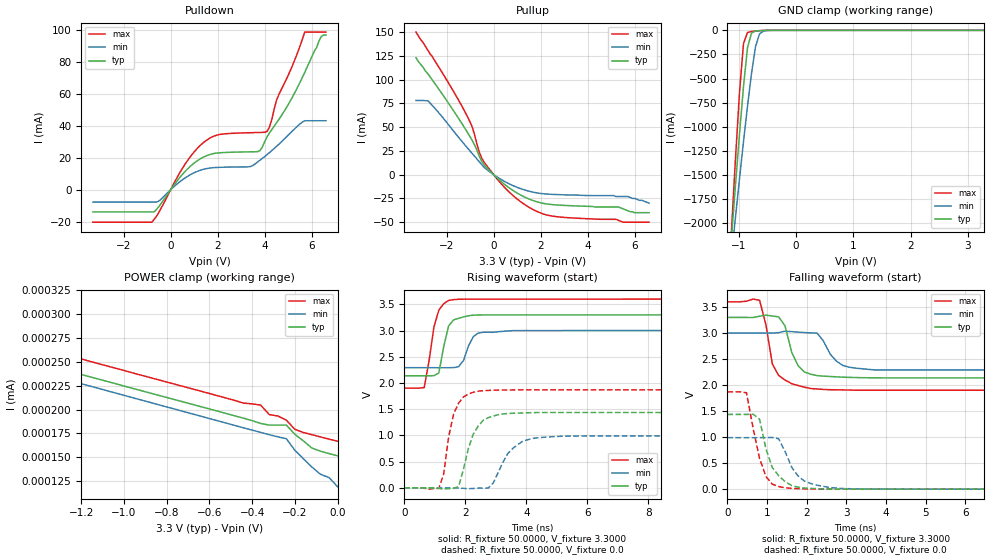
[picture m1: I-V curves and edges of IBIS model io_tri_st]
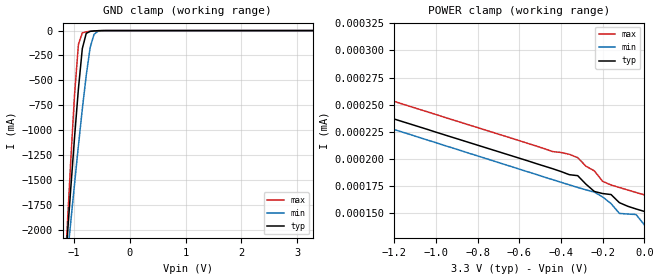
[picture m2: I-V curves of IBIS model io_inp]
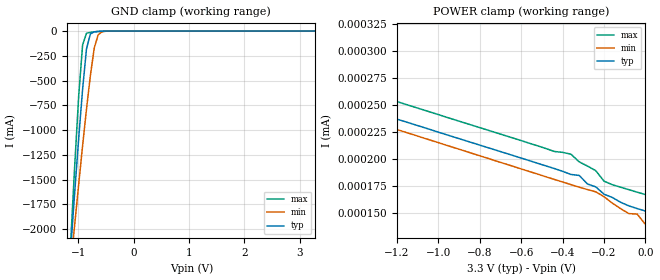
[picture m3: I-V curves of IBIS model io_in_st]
[IBIS ver] 3.2
[File name] sps1616.ibs
[File Rev] 1.3
[Date]  16 Jan 2014
[Source] Integrated Device Techology, Inc. (IDT)
[Disclaimer]
   Integrated Device Technology, Inc. ("IDT") hereby grants the
   user of this IBIS model a non-exclusive, nontransferable
   license to use this IBIS model under the following terms. The
   user is granted this license only to use the IBIS model and is
   not granted rights to sell, copy (except as needed to run the
   IBIS model), rent, lease or sub-license the IBIS model in
   whole or in part, or in modified form to anyone. The User may
   modify the IBIS model to suit its specific applications, but
   rights to derivative works and such modifications shall belong
   to IDT. This IBIS model is provided on an AS IS" basis and IDT
   makes absolutely no warranty with respect to the information
   contained herein. IDT DISCLAIMS AND CUSTOMER WAIVES ALL
   WARRANTIES, EXPRESS AND IMPLIED, INCLUDING WARRANTIES OF
   MERCHANTABILITY AND FITNESS FOR A PARTICULAR PURPOSE. THE
   ENTIRE RISK AS TO QUALITY AND PERFORMANCE IS WITH THE USER
   ACCORDINGLY, IN NO EVENT SHALL IDT BE LIABLE FOR ANY DIRECT OR
   INDIRECT DAMAGES, WHETHER IN CONTRACT OR TORT, INCLUDING ANY
   LOST PROFITS OR OTHER INCIDENTAL, CONSEQUENTIAL, EXEMPLARY, OR
   PUNITIVE DAMAGES ARISING OUT OF THE USE OR APPLICATION OF THE
   IBIS model. Further, IDT reserves the right to make changes
   without notice to any product herein to improve reliability,
   function, or design. IDT does not convey any license under
   patent rights or any other intellectual property rights,
   including those of third parties. IDT is not obligated to
   provide maintenance or support for the licensed IBIS model.
[Copyright] Copyright 2012, IDT, All Rights Reserved.
[Notes]
*******************Revision History***************************************
Revision 1.3: 16 Jan 2014 : Added individual pin parasitic information
|   Component SPS1616_slowio
[Component] SPS1616_slowio
[Manufacturer] Integrated Device Techology, Inc.
[Package]
| variable   typ   min   max
R_pkg   0.506   0.188   0.752
L_pkg   4.84nH   2.30nH   6.89nH
C_pkg   2.32pF   1.67pF   2.76pF
[Pin]  signal_name   model_name   R_pin   L_pin   C_pin
A17   id6   io_inp   0.73675   6.41E-09   2.53E-12
A18   sda   io_tri_st   0.65663   6.16E-09   2.58E-12
A19   scl   io_tri_st   0.735   6.86E-09   2.70E-12
A2   tms   io_in_pu   0.6938   6.41E-09   2.64E-12
B1   tdo   io_tri_outp   0.68057   6.41E-09   2.65E-12
B17   id7   io_inp   0.619   5.51E-09   2.26E-12
B18   id2   io_inp   0.57434   5.54E-09   2.40E-12
B19   id1   io_inp   0.58321   5.70E-09   2.55E-12
B2   tck   io_in_st   0.69135   6.48E-09   2.68E-12
B20   id0   io_inp   0.75241   6.89E-09   2.75E-12
C1   tdi   io_in_pu   0.61721   5.79E-09   2.54E-12
C17   id8   io_inp   0.47421   4.54E-09   2.27E-12
C18   id5   io_inp   0.57865   5.50E-09   2.49E-12
C19   id4   io_inp   0.635   5.98E-09   2.53E-12
C2   trst_n   io_in_st_pu   0.56042   5.30E-09   2.34E-12
C20   id3   io_inp   0.70895   6.56E-09   2.76E-12
D1   irq_n   io_tri_outp   0.56524   5.34E-09   2.45E-12
D16   mm_n   io_in_pu   0.44876   4.51E-09   2.15E-12
D17   id9   io_inp   0.44456   4.60E-09   2.10E-12
E10   pd2   io_in_pu   0.37216   3.85E-09   2.12E-12
E11   pd1   io_in_pu   0.33843   3.88E-09   2.04E-12
E12   pd0   io_in_pu   0.40125   4.71E-09   2.41E-12
E16   ads   io_inp   0.36136   3.93E-09   2.06E-12
E9   pd3   io_in_pu   0.30714   3.18E-09   2.00E-12
J16   pd15   io_in_pu   0.26698   2.98E-09   1.82E-12
J5   pd8   io_in_pu   0.19421   2.32E-09   1.67E-12
K16   pd14   io_in_pu   0.25759   2.90E-09   1.77E-12
K5   pd9   io_in_pu   0.29585   3.48E-09   1.83E-12
L16   pd13   io_in_pu   0.18822   2.30E-09   1.72E-12
L5   pd10   io_in_pu   0.41991   4.13E-09   2.30E-12
M16   pd12   io_in_pu   0.23133   2.32E-09   1.81E-12
M5   pd11   io_in_pu   0.33402   3.60E-09   1.91E-12
T10   pd5   io_in_pu   0.3759   3.58E-09   2.00E-12
T11   pd10   io_in_pu   0.31528   3.20E-09   1.92E-12
T12   pd7   io_in_pu   0.19723   2.50E-09   1.85E-12
T5   qcfg1   io_tri_in   0.39577   3.80E-09   2.14E-12
T9   pd4   io_in_pu   0.3506   3.98E-09   2.56E-12
U4   qcfg0   io_tri_in   0.46727   4.29E-09   2.23E-12
U5   qcfg2   io_tri_in   0.44778   4.16E-09   2.18E-12
V1   mrst_n   io_in_st   0.6805   5.96E-09   2.70E-12
V19   spd0   io_inp   0.62204   5.43E-09   2.61E-12
V4   qcfg3   io_tri_in   0.48643   4.32E-09   2.33E-12
W1   qcfg4   io_tri_in   0.73005   6.25E-09   2.74E-12
W19   spd1   io_inp   0.62846   5.93E-09   2.49E-12
W2   qcfg5   io_tri_in   0.60658   5.21E-09   2.47E-12
W20   spd2   io_inp   0.70495   6.45E-09   2.60E-12
W3   qcfg6   io_tri_in   0.56254   4.96E-09   2.40E-12
W4   qcfg7   io_tri_in   0.50075   4.51E-09   2.33E-12
Y2   mcast   io_in_st   0.69157   6.08E-09   2.73E-12
Y3   fsel0   io_in_pu   0.69351   6.37E-09   2.68E-12
Y4   fsel1   io_in_pu   0.61581   5.67E-09   2.54E-12
V20   ref_clk_p  refclkin   0.60259   5.13E-09   1.90E-12
U20   ref_clk_n  refclkin   0.58152   4.95E-09   1.85E-12
| Models and submodels in the file (8): io_tri_st (I/O), io_inp (Input), io_in_st (Input), io_tri_outp (3-state), io_in_st_pu (Input), io_in_pu (Input), io_tri_in (I/O), refclkin (Terminator)
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|   Model io_tri_st
[Model]  io_tri_st
Model_type I/O
Polarity   Non-Inverting
Enable   Active-Low
Vinl =   0.8000V
Vinh =   2.0000V
Vmeas =  1.6500V
Cref =   50.0000pF
Rref =   1.0000M
Vref =   0.0V
C_comp   2.4706pF   2.4445pF   2.5092pF
[Temperature Range]   25.0000   0.1250k   -40.0000
[Voltage Range]   3.3000V   3.0000V   3.6000V
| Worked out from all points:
|   slope of the pulldown table from 0 to 0.495 V, typ, clamps not added: 51.9 ohm
|   slope of the pullup table from 0 to 0.495 V, typ, clamps not added: 45.6 ohm
|   GND clamp passes 1 mA (typ) near -0.54 V on its own axis
|   POWER clamp passes 1 mA (typ) near -2.49 V on its own axis
|   rising waveform, R_fixture 50.0000, V_fixture 3.3000: 20-80 % time 255ps typ, 295ps min, 313ps max; typ from 2.14 V to 3.3 V
|   rising waveform, R_fixture 50.0000, V_fixture 0.0: 20-80 % time 484ps typ, 645ps min, 366ps max; typ from 0 V to 1.44 V
|   falling waveform, R_fixture 50.0000, V_fixture 3.3000: 20-80 % time 312ps typ, 393ps min, 314ps max; typ from 3.3 V to 2.14 V
|   falling waveform, R_fixture 50.0000, V_fixture 0.0: 20-80 % time 397ps typ, 462ps min, 342ps max; typ from 1.44 V to 0 V
[Pulldown]
|Voltage   I(typ)   I(min)   I(max)
-3.3V     -13.86mA   -7.71mA    -20.29mA
-800mV    -13.86mA   -7.71mA    -20.29mA
600mV     11.25mA    7.285mA    15.72mA
1.4V      20.53mA    12.85mA    29.63mA
2.1V      23.2mA     14.09mA    34.69mA
3.4V      23.8mA     14.57mA    35.78mA
3.8V      24.57mA    18.57mA    35.93mA
4.2V      35.62mA    23.3mA     39.28mA
4.5V      41.93mA    27.2mA     56.15mA
5.7V      73.6mA     43.26mA    98.81mA
6.4V      96mA       43.26mA    98.81mA
6.6V      97mA       43.26mA    98.81mA
[Pullup]
|Voltage   I(typ)   I(min)   I(max)
-3.3V     123mA      78.1mA     150mA
-2.8V     106.3mA    77.79mA    131mA
-1.2V     47.86mA    30.59mA    65.19mA
-900mV    35.42mA    21.89mA    49.37mA
-500mV    13.73mA    10.33mA    16.95mA
300mV     -6.88mA    -4.819mA   -8.986mA
1V        -19.4mA    -13.37mA   -25.69mA
1.7V      -27.44mA   -18.53mA   -37.02mA
2.4V      -31.25mA   -20.6mA    -43.2mA
5.3V      -34mA      -23mA      -48mA
5.7V      -38mA      -23mA      -50mA
6.6V      -40mA      -30mA      -50mA
[GND_clamp]
|Voltage   I(typ)   I(min)   I(max)
-3.3V     -20.24A    -15.41A    -26.98A
-1.13V    -2.159A    -2.344A    -2.077A
-1.06V    -1.611A    -1.941A    -1.338A
-990mV    -1.08A     -1.545A    -651.6mA
-920mV    -586.7mA   -1.158A    -139.4mA
-850mV    -181.3mA   -789.1mA   -22.48mA
-780mV    -28.37mA   -450.9mA   -12.35mA
-710mV    -7.599mA   -171.5mA   -7.64mA
-640mV    -3.504mA   -37.73mA   -3.899mA
-570mV    -1.414mA   -7.386mA   -1.365mA
-360mV    -3.781uA   -39.23uA   -907.8nA
3.28V     150.3nA    221.4nA    148.8nA
[POWER_clamp]
|Voltage   I(typ)   I(min)   I(max)
-3.28V    3.127A     1.353A     6.658A
-2.28V    531.3nA    314.4nA    683.5uA
-2.24V    350.6nA    298.4nA    96.38uA
-2.12V    294.9nA    284.6nA    571.2nA
-2.04V    289.2nA    279.3nA    310.9nA
-1.44V    251.4nA    241.7nA    267.6nA
-360mV    185.4nA    176nA      204.6nA
-320mV    183.7nA    173.6nA    194.7nA
-240mV    183.7nA    169.4nA    188.9nA
-200mV    174nA      157.3nA    179.2nA
-120mV    159.6nA    139.7nA    173.6nA
0V        151.5nA    119.1nA    166.8nA
[Ramp]
| variable   typ   min   max
dV/dt_r  0.8616/0.4836n   0.5939/0.6346n   1.1214/0.3563n
dV/dt_f  0.6978/0.3030n   0.4254/0.3829n   1.0188/0.3144n
R_load = 50.0000
[Rising Waveform]
R_fixture= 50.0000
V_fixture= 3.3000
V_fixture_min= 3.0000
V_fixture_max= 3.6000
L_fixture= 0.0H
C_fixture= 0.0F
|time   V(typ)   V(min)   V(max)
0s        2.137V     2.291V     1.902V
650ps     2.137V     2.291V     1.912V
970ps     2.139V     2.291V     3.069V
1.13ns    2.19V      2.29V      3.39V
1.45ns    3.088V     2.29V      3.575V
1.78ns    3.233V     2.312V     3.596V
1.94ns    3.26V      2.431V     3.598V
2.26ns    3.293V     2.886V     3.599V
2.59ns    3.297V     2.967V     3.599V
16ns      3.3V       3V         3.6V
[Rising Waveform]
R_fixture= 50.0000
V_fixture= 0.0
V_fixture_min= 0.0
V_fixture_max= 0.0
L_fixture= 0.0H
C_fixture= 0.0F
|time   V(typ)   V(min)   V(max)
0s        2.775uV    3.203uV    2.534uV
1.13ns    -8.225mV   55.74uV    -11.75mV
1.29ns    -25.06mV   29.84uV    267.8mV
1.62ns    -9.675mV   -1.142mV   1.421V
1.78ns    25.34mV    -3.25mV    1.617V
2.42ns    1.18V      -5.263mV   1.844V
2.91ns    1.367V     93.16mV    1.862V
3.56ns    1.422V     755mV      1.867V
4.36ns    1.436V     954.3mV    1.869V
16ns      1.436V     989.8mV    1.869V
[Falling Waveform]
R_fixture= 50.0000
V_fixture= 3.3000
V_fixture_min= 3.0000
V_fixture_max= 3.6000
L_fixture= 0.0H
C_fixture= 0.0F
|time   V(typ)   V(min)   V(max)
0s        3.3V       3V         3.6V
810ps     3.323V     3V         3.629V
970ps     3.343V     2.999V     3.16V
1.13ns    3.328V     3V         2.409V
1.29ns    3.311V     3.007V     2.186V
1.78ns    2.374V     3.018V     1.992V
2.1ns     2.209V     3.003V     1.934V
2.91ns    2.152V     2.376V     1.907V
3.72ns    2.14V      2.291V     1.902V
16ns      2.137V     2.291V     1.902V
[Falling Waveform]
R_fixture= 50.0000
V_fixture= 0.0
V_fixture_min= 0.0
V_fixture_max= 0.0
L_fixture= 0.0H
C_fixture= 0.0F
|time   V(typ)   V(min)   V(max)
0s        1.436V     989.8mV    1.869V
480ps     1.436V     989.8mV    1.853V
810ps     1.343V     989.7mV    589.1mV
1.13ns    416.7mV    992.8mV    96.68mV
1.29ns    259.7mV    969.6mV    49.13mV
1.45ns    146.7mV    726.9mV    26.57mV
1.62ns    69.81mV    420.8mV    15.73mV
1.94ns    22.55mV    154.2mV    5.519mV
2.91ns    1.17mV     12.07mV    315.6uV
16ns      -16.86uV   0V         -8.252uV
|   Model io_inp
[Model]  io_inp
Model_type Input
Polarity   Non-Inverting
Vinl =   0.8000V
Vinh =   2.0000V
C_comp   2.5537pF   2.5182pF   2.6032pF
[Temperature Range]   25.0000   0.1250k   -40.0000
[Voltage Range]   3.3000V   3.0000V   3.6000V
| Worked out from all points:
|   GND clamp passes 1 mA (typ) near -0.54 V on its own axis
|   POWER clamp passes 1 mA (typ) near -2.49 V on its own axis
[GND_clamp]
|Voltage   I(typ)   I(min)   I(max)
-3.3V     -20.24A    -15.41A    -26.98A
-1.13V    -2.159A    -2.344A    -2.077A
-1.06V    -1.611A    -1.941A    -1.338A
-990mV    -1.08A     -1.545A    -651.6mA
-920mV    -586.7mA   -1.158A    -139.4mA
-850mV    -181.3mA   -789.1mA   -22.48mA
-780mV    -28.37mA   -450.9mA   -12.35mA
-710mV    -7.599mA   -171.5mA   -7.64mA
-640mV    -3.504mA   -37.73mA   -3.899mA
-570mV    -1.414mA   -7.386mA   -1.365mA
-360mV    -3.781uA   -39.23uA   -907.8nA
3.28V     150.3nA    331.4nA    148.8nA
[POWER_clamp]
|Voltage   I(typ)   I(min)   I(max)
-3.28V    3.127A     1.353A     6.658A
-2.28V    531.3nA    314.4nA    683.5uA
-2.2V     310nA      291.6nA    13.72uA
-2.16V    299.2nA    287.6nA    2.182uA
-2.08V    291.9nA    281.9nA    344.7nA
-1.72V    268.7nA    259nA      285.1nA
-320mV    184.5nA    173.6nA    201.1nA
-240mV    169.9nA    169.3nA    188.9nA
-200mV    168nA      164.8nA    179.2nA
-120mV    159.6nA    149.7nA    173.6nA
-40mV     153.8nA    148.7nA    169nA
0V        151.5nA    139.1nA    166.8nA
|   Model io_in_st
[Model]  io_in_st
Model_type Input
Polarity   Non-Inverting
Vinl =   0.8000V
Vinh =   2.0000V
C_comp   2.5537pF   2.5183pF   2.6032pF
[Temperature Range]   25.0000   0.1250k   -40.0000
[Voltage Range]   3.3000V   3.0000V   3.6000V
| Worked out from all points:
|   GND clamp passes 1 mA (typ) near -0.54 V on its own axis
|   POWER clamp passes 1 mA (typ) near -2.49 V on its own axis
[GND_clamp]
|Voltage   I(typ)   I(min)   I(max)
-3.3V     -20.24A    -15.41A    -26.98A
-1.13V    -2.159A    -2.344A    -2.077A
-1.06V    -1.611A    -1.941A    -1.338A
-990mV    -1.08A     -1.545A    -651.6mA
-920mV    -586.7mA   -1.158A    -139.4mA
-850mV    -181.3mA   -789.1mA   -22.48mA
-780mV    -28.37mA   -450.9mA   -12.35mA
-710mV    -7.599mA   -171.5mA   -7.64mA
-640mV    -3.504mA   -37.73mA   -3.899mA
-570mV    -1.414mA   -7.386mA   -1.365mA
-360mV    -3.781uA   -39.23uA   -907.8nA
3.28V     150.3nA    176.4nA    148.8nA
[POWER_clamp]
|Voltage   I(typ)   I(min)   I(max)
-3.28V    3.127A     1.353A     6.658A
-2.28V    531.3nA    314.4nA    683.5uA
-2.24V    350.6nA    298.4nA    96.38uA
-2.2V     310nA      291.6nA    13.72uA
-2.16V    299.2nA    287.6nA    2.182uA
-2.08V    291.9nA    281.9nA    344.7nA
-1.72V    268.7nA    259nA      285.1nA
-360mV    185.4nA    176nA      204.2nA
-240mV    173.9nA    169.3nA    188.9nA
-200mV    167.1nA    164.8nA    179.2nA
-40mV     153.8nA    148.7nA    169nA
0V        151.5nA    139.1nA    166.8nA
